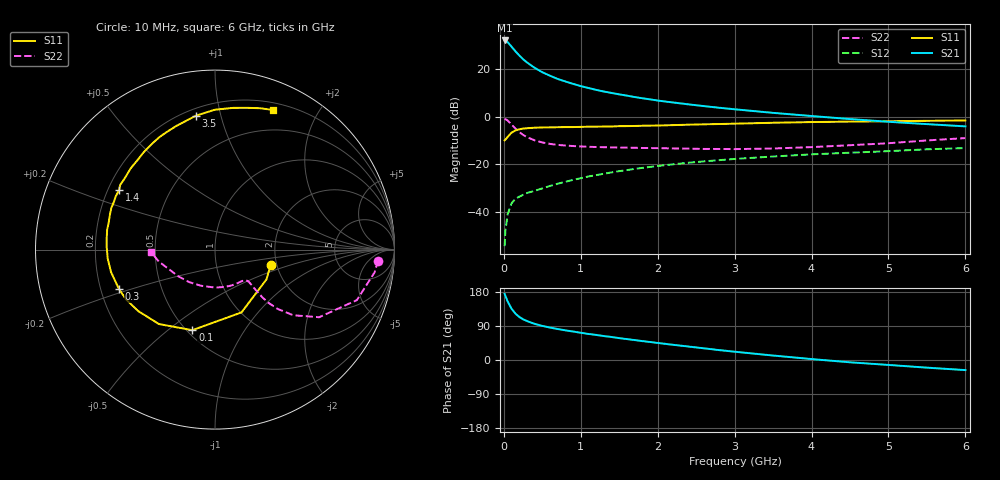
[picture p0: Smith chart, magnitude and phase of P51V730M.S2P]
! SIEMENS Small Signal Semiconductors
! BFP183
! Si NPN RF Bipolar Junction Transistor in SOT143
! VCE = 1.75 V  IC = 30 mA
! Common Emitter S-Parameters:  March  1996
# GHz  S  MA  R  50
!  f  S11  S21  S12  S22
! GHz  MAG  ANG  MAG  ANG  MAG  ANG  MAG  ANG
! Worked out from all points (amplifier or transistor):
!   36 points, 10 MHz to 6 GHz, reference 50 ohm
!   highest |S21| = 32.2 dB at 10 MHz (marker M1)
!   |S21| within 3 dB of that: start of sweep to 110 MHz
!   unconditionally stable (mu >= 1): 466.1 MHz to end of sweep
!   at 250 MHz: K = 0.70, MSG = 28.5 dB, |S12| = -32.8 dB
!   at 1.4 GHz: K = 1.30, MAG = 13.5 dB, |S12| = -23.4 dB
!   at 6 GHz: K = 1.03, MAG = 3.5 dB, |S12| = -13.1 dB
!   S11 on the Smith chart (normalised r, x): 10 MHz: 1.86, -0.35; 100 MHz: 0.53, -0.61; 300 MHz: 0.28, -0.18; 1.4 GHz: 0.25, +0.27; 3.5 GHz: 0.24, +0.84; 6 GHz: 0.27, +1.47
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0.01  0.3221 -15.4  40.72 174.6  0.0019 81.7  0.9106 -3.9
0.02  0.3313 -30.1  40.41 169.5  0.004 75.3  0.8983 -8.1
0.05  0.3798 -67.1  37.52 154.3  0.009 73.6  0.8389 -19.6
0.1  0.4663 -105.7  30.12 135.3  0.0152 56.8  0.6919 -33.0
0.15  0.5192 -127.0  24.17 122.5  0.0189 51.4  0.5693 -40.0
0.2  0.5481 -141.3  19.68 113.8  0.0209 50.2  0.4814 -43.4
0.25  0.568 -150.8  16.4 107.4  0.0229 48.7  0.419 -44.9
0.3  0.5782 -157.6  14.07 102.8  0.025 49.0  0.3756 -45.2
0.4  0.5925 -167.7  10.83 95.4  0.0278 50.8  0.3216 -44.8
0.5  0.6 -175.3  8.713 90.0  0.0313 51.4  0.2898 -44.2
0.6  0.6033 178.8  7.375 85.6  0.0352 54.4  0.2704 -43.8
0.7  0.6069 173.7  6.306 81.7  0.0392 56.0  0.258 -43.7
0.8  0.6111 169.5  5.576 78.2  0.043 56.4  0.2497 -44.1
1.1  0.6225 158.1  4.061 68.7  0.0558 57.7  0.235 -47.0
1.4  0.6287 148.2  3.196 60.7  0.0679 56.9  0.2282 -51.9
1.8  0.6517 136.5  2.475 49.9  0.0846 54.7  0.2219 -60.2
2.2  0.6719 126.4  2.014 40.1  0.1005 51.2  0.2168 -70.1
2.8  0.7085 112.1  1.56 26.1  0.123 45.5  0.2115 -88.1
3.5  0.7532 98.2  1.217 11.8  0.1468 39.0  0.2162 -111.4
4.5  0.7961 82.7  0.901 -6.1  0.1764 29.4  0.2537 -144.4
5.5  0.8271 72.2  0.705 -20.2  0.208 20.9  0.3199 -168.0
6  0.8428 67.3  0.632 -26.6  0.2209 16.1  0.3584 -178.1
